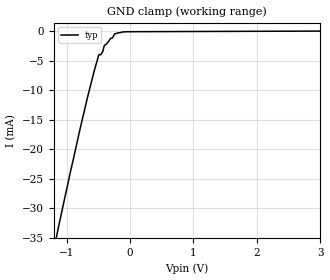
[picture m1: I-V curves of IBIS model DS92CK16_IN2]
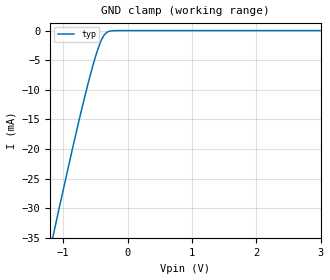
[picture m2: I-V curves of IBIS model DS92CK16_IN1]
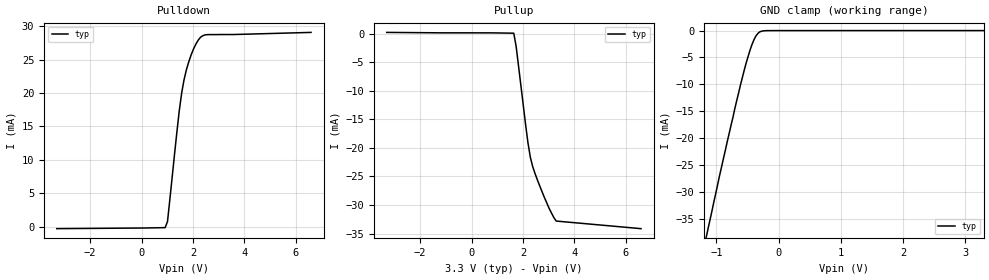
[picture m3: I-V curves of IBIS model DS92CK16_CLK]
|   National Semiconductor Corporation
|   Interface Products Group
|   IBIS Model of DS92CK16TMTC
|   24 Pin TSSOP Package
[IBIS Ver]   2.1
[Comment char]  |_char
[File name]   92ck16.ibs
[File Rev]   1.0
[Date]   11/15/2000
[Source]   File originated at National Semiconductor Corporation.
   Interface Group/Analog Division. All data based on
   HSPICE simulation.Sim generated by milt
[Notes]   File created/verfied by milt.
   92lv090a.ibs used as template
   11/15  CLKout Voh table modified so Vtable=Vcc-Vmeas.
[Disclaimer]
(C) Copyright National Semiconductor Corporation 1994
   All rights reserved
   National Semiconductor Corporation hereby grants
the user of this IBIS model a non-exclusive, nontransferable
license to use this IBIS model under the following terms.
Before using this IBIS model, the user should read this
license.  If the user does not accept these terms,  the
IBIS model should be returned to National within 30 days.
   The user is granted this license only to use the
IBIS model and is not granted rights to sell, load, rent,
lease or license the IBIS model in whole or in part, or in
modified form to anyone other than user. User may modify
the IBIS model to suit its specific applications but rights
to derivative works and such modifications shall belong to
National.
   This IBIS model is provided on an "AS IS" basis and
National makes absolutely no warranty with respect to the
information contained herein.NATIONAL DISCLAIMS AND CUSTOMER
WAIVES ALL WARRANTIES, EXPRESS OR IMPLIED, INCLUDING
WARRANTIES OF MERCHANTABILITY OR FITNESS FOR A PARTICULAR
PURPOSE. The entire risk as to quality and performance is
with the Customer. ACCORDINGLY, IN NO EVENT SHALL THE
COMPANY BE LIABLE FOR ANY DAMAGES, WHETHER IN CONTRACT OR
TORT,INCLUDING ANY LOST PROFITS OR OTHER INCIDENTAL,
CONSEQUENTIAL, EXEMPLARY, OR PUNITIVE DAMAGES ARISING OUT
OF THE USE OR APPLICATION OF THE IBIS model provided in
this package.Further, National reserves the right to make
changes without notice to any product herein to improve
reliability, function, or design. National does not convey
any license under patent rights or any other intellectual
property rights, including those of third parties.
   National is not obligated to provide maintenance or support
for the licensed IBIS model.
Contact National at ATTN:INTERFACE APPLICATIONS/IBIS MODELS.
2900 Semiconductor Drive, M/S A2595, Santa Clara, CA 95052-8090
[Copyright]   Copyright 1994, National Semiconductor, All Rights Reserved
[Component]   DS92CK16
[Manufacturer]  National Semiconductor Corp
[Package]
|   typ   min   max
R_pkg   50.0m   NA   NA
L_pkg   0.542n   NA   NA
C_pkg   0.967p   NA   NA
[Pin]   signal_name  model_name   R_pin   L_pin   C_pin
1   GND   GND   50.0m   1.06n   0.16p
2   OE   DS92CK16_IN1   50.0m   0.80n   0.17p
3   NC   NC   50.0m   0.54n   0.12p
4   VCCA   POWER   50.0m   0.28n   0.06p
5   GNDA   GND   50.0m   0.28n   0.03p
6   CLKI/O+   DS92CK16_CLK   50.0m   0.29n   0.04p
7   CLKI/O-   DS92CK16_CLK   50.0m   0.29n   0.04p
8   GNDA   GND   50.0m   0.28n   0.03p
9   CrdCLKin   DS92CK16_IN2   50.0m   0.28n   0.06p
10   NC   NC   50.0m   0.54n   0.12p
11   DE   DS92CK16_IN1   50.0m   0.80n   0.17p
12   GND   GND   50.0m   1.06n   0.16p
13   CLKout5   DS92CK16_COUT   50.0m   1.06n   0.16p
14   GND   GND   50.0m   0.80n   0.17p
15   CLKout4   DS92CK16_COUT   50.0m   0.54n   0.12p
16   VCC   POWER   50.0m   0.28n   0.06p
17   CLKout3   DS92CK16_COUT   50.0m   0.28n   0.03p
18   GND   GND   50.0m   0.29n   0.04p
19   CLKout2   DS92CK16_COUT   50.0m   0.29n   0.04p
20   DVCC   POWER   50.0m   0.28n   0.03p
21   CLKout1   DS92CK16_COUT   50.0m   0.28n   0.06p
22   GND   GND   50.0m   0.54n   0.12p
23   CLKout0   DS92CK16_COUT   50.0m   0.80n   0.17p
24   VCC   POWER   50.0m   1.06n   0.16p
[Diff_pin]   inv_pin   vdiff   tdelay_typ   tdelay_min   tdelay_max
| The '+' pin is Diff_pin and the '-' pin is the inv_pin
6   7   0.100   0 0 0
| Models and submodels in the file (4): DS92CK16_IN2 (Input), DS92CK16_IN1 (Input), DS92CK16_CLK (I/O), DS92CK16_COUT (Output)
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|   CrdCLK Input  MODEL
[Model]   DS92CK16_IN2
Model_type   Input
|Signals   CrdCLKin
Vinh = 2.0
Vinl = 0.8
|   typ   min   max
C_comp   5.18pF   NA   NA
|   typ   min   max
[Temperature Range]   25.0   NA   NA
[Voltage range]   3.3V   NA   NA
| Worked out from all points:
|   GND clamp passes 1 mA (typ) near -0.27 V on its own axis
[Power_clamp]
| Note that the[POWER_clamp]voltage table is referenced to Vcc
| and is calculated using Vtable=Vcc - Vmeasured.
| Driver inputs do not have power clamp
|Voltage   I(typ)   I(min)   I(max)
-3.3V     0A         NA         NA
3.3V      0A         NA         NA
[GND_clamp]
|Voltage   I(typ)   I(min)   I(max)
-3.3V     -126mA     NA         NA
-1.133V   -33.56mA   NA         NA
-797mV    -17.08mA   NA         NA
-552mV    -6.281mA   NA         NA
-490mV    -3.998mA   NA         NA
-459mV    -3.989mA   NA         NA
-429mV    -3.472mA   NA         NA
-405mV    -2.448mA   NA         NA
-276mV    -1.184mA   NA         NA
-244mV    -496.9uA   NA         NA
-62mV     -111.1uA   NA         NA
3V        25.3nA     NA         NA
|   Driver  Enable, Output EnabLE MODEL
[Model]   DS92CK16_IN1
Model_type   Input
|Signals   DE,OE
Vinh = 2.0
Vinl = 0.8
|   typ   min   max
C_comp   5.38pF   NA   NA
|   typ   min   max
[Temperature Range]   25.0   NA   NA
[Voltage range]   3.3V   NA   NA
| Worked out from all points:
|   GND clamp passes 1 mA (typ) near -0.38 V on its own axis
[GND_clamp]
|   Voltage   I(typ)   I(min)   I(max)
-3.3V     -282A      NA         NA
-1.163V   -35.05mA   NA         NA
-1.133V   -33.51mA   NA         NA
-949mV    -24.46mA   NA         NA
-766mV    -15.74mA   NA         NA
-582mV    -7.649mA   NA         NA
-490mV    -4.136mA   NA         NA
-429mV    -2.198mA   NA         NA
-368mV    -836.6uA   NA         NA
-306mV    -201.3uA   NA         NA
-122mV    -1.572uA   NA         NA
3V        25.31nA    NA         NA
[Power_clamp]
| Note that the[POWER_clamp]voltage table is referenced to Vcc
| and is calculated using Vtable=Vcc - Vmeasured.
| Driver Enable input has no Power Clamp
|Voltage   I(typ)   I(min)   I(max)
-3.3V     0A         NA         NA
3.3V      0A         NA         NA
|   BLVDS CLKI/O  Output  MODEL
[Model]   DS92CK16_CLK
Model_type   I/O
| Signals   CLKI/O  These signals are TRI-STATE type
Vmeas = 1.2V   |This is 0.0v differential on ouput
Cref = 5pF   |Timing specification test load capacitance value
Rref = 57   |Note: 57 Ohm between the two driver outputs
Vref = 1.2   |Timing specification test load voltage; GND
Vinl = 0.8
Vinh = 2.0
| variable   typ   min   max
C_comp   7.21pF   NA   NA
|   typ   min   max
[Temperature Range]   25.0   NA   NA
[Voltage range]   3.3V   NA   NA
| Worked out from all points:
|   slope of the pulldown table from 0 to 0.495 V, typ, clamps not added: 15.7 kohm
|   GND clamp passes 1 mA (typ) near -0.36 V on its own axis
[Pulldown]
|   Voltage   I(typ)   I(min)   I(max)
-3.3V     -313uA     NA         NA
920mV     -158.8uA   NA         NA
1.012V    752.2uA    NA         NA
1.379V    14.22mA    NA         NA
1.471V    17.38mA    NA         NA
1.564V    20.02mA    NA         NA
1.654V    21.96mA    NA         NA
1.839V    24.68mA    NA         NA
2.022V    26.59mA    NA         NA
2.206V    27.93mA    NA         NA
2.574V    28.77mA    NA         NA
6.6V      29.1mA     NA         NA
[Pullup]
| Note that the[Pullup]voltage table is referenced to Vcc
| and is calculated using Vtable=Vcc - Vmeasured.
|   Voltage   I(typ)   I(min)   I(max)
-3.3V     248uA      NA         NA
1.645V    106.9uA    NA         NA
1.738V    -2.223mA   NA         NA
2.104V    -15.85mA   NA         NA
2.197V    -19.07mA   NA         NA
2.289V    -21.6mA    NA         NA
2.38V     -23.23mA   NA         NA
2.564V    -25.59mA   NA         NA
3.023V    -30.6mA    NA         NA
3.208V    -32.22mA   NA         NA
3.299V    -32.81mA   NA         NA
6.6V      -34.14mA   NA         NA
[GND_clamp]
| CLKI/O outputs in TRI-STATE.
|   Voltage   I(typ)   I(min)   I(max)
-3.3V     -17.51A    NA         NA
-1.164V   -38.38mA   NA         NA
-1.133V   -36.73mA   NA         NA
-950mV    -26.96mA   NA         NA
-706mV    -14.58mA   NA         NA
-522mV    -6.021mA   NA         NA
-460mV    -3.637mA   NA         NA
-398mV    -1.737mA   NA         NA
-368mV    -1.058mA   NA         NA
-307mV    -271uA     NA         NA
-153mV    -8.911uA   NA         NA
3.3V      0A         NA         NA
[POWER_clamp]
| Note that the[POWER_clamp]voltage table is referenced to Vcc
| and is calculated using Vtable=Vcc - Vmeasured.
| Outputs in Tri-state.
|Voltage   I(typ)   I(min)   I(max)
-3.3V     0A         NA         NA
3.3V      0A         NA         NA
[Ramp]
| Note: Ramp rate measured on single-ended Driver Output.
|   typ   min   max
dV/dt_r   250m/225p   314m/234p   218m/223p
dV/dt_f   250m/289p   314m/358p   218m/215p
R_load = 37Ohm | Note: This 37 Ohm is across the two driver output
